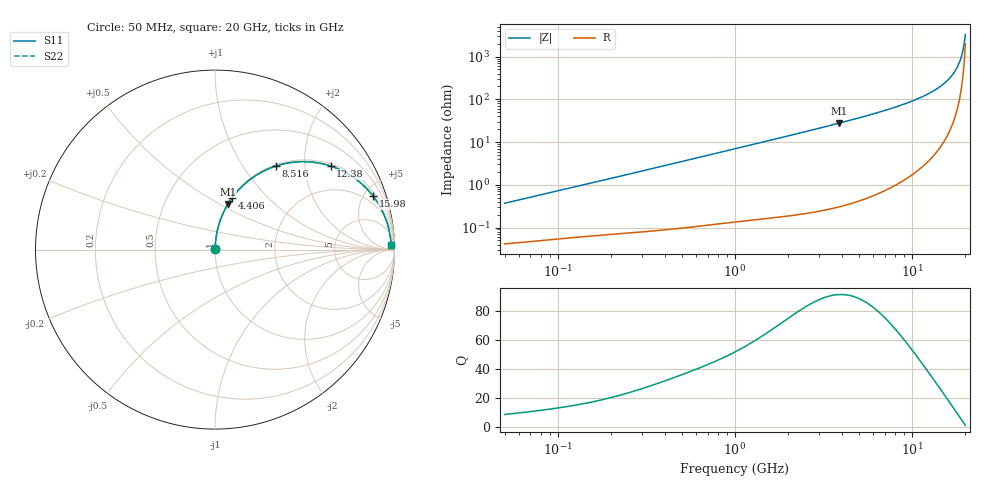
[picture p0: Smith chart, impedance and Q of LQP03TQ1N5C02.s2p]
!Murata Part Number: LQP03TQ1N5C02
!These Parameters are Measured in Series Mode Connection
!  o--[Z]--o
!Port1  Port2
!  o-------o
!Freq. Start=50[MHz] Stop=20[GHz], 401[Steps]
# Hz S RI R 50
!Freq.(Hz) S11(Real) S11(Imag) S21(Real) S21(Imag) S12(Real) S12(Imag) S22(Real) S22(Imag)
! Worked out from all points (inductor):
!   401 points, 50 MHz to 20 GHz, reference 50 ohm
!   read as one part in series: L = 1.16 nH near 51.52 MHz
!   highest Q = 91.2 at 3.85 GHz (marker M1), where L = 1.14 nH
!   S11 on the Smith chart (normalised r, x): 50 MHz: 1.00, +0.01; 4.406 GHz: 1.01, +0.64; 8.516 GHz: 1.02, +1.43; 12.38 GHz: 1.07, +2.71; 15.98 GHz: 1.31, +5.74; 20 GHz: 40, +53
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5e7  0.000427 0.00367  0.9996 -0.00367  0.9996 -0.00367  0.000427 0.00367
1.364002e8  0.000701 0.00973  0.9993 -0.00973  0.9993 -0.00973  0.000701 0.00973
3.721004e8  0.00154 0.0261  0.9985 -0.0261  0.9985 -0.0261  0.00154 0.0261
1e9  0.00616 0.0692  0.9938 -0.0692  0.9938 -0.0692  0.00616 0.0692
1.714689e9  0.0158 0.1175  0.9842 -0.1175  0.9842 -0.1175  0.0158 0.1175
2.728004e9  0.0376 0.1844  0.9624 -0.1844  0.9624 -0.1844  0.0376 0.1844
3.850025e9  0.0731 0.2549  0.9269 -0.2549  0.9269 -0.2549  0.0731 0.2549
4.405649e9  0.0951 0.2879  0.9049 -0.2879  0.9049 -0.2879  0.0951 0.2879
5.856089e9  0.1657 0.3659  0.8343 -0.3659  0.8343 -0.3659  0.1657 0.3659
7.442007e9  0.2632 0.4335  0.7368 -0.4335  0.7368 -0.4335  0.2632 0.4335
8.516016e9  0.3393 0.4657  0.6607 -0.4657  0.6607 -0.4657  0.3393 0.4657
1.050288e10  0.4943 0.49  0.5057 -0.49  0.5057 -0.49  0.4943 0.49
1.238412e10  0.6447 0.4656  0.3553 -0.4656  0.3553 -0.4656  0.6447 0.4656
1.417136e10  0.7748 0.4001  0.2252 -0.4001  0.2252 -0.4001  0.7748 0.4001
1.597544e10  0.8794 0.3001  0.1206 -0.3001  0.1206 -0.3001  0.8794 0.3001
1.721783e10  0.9308 0.2182  0.0692 -0.2182  0.0692 -0.2182  0.9308 0.2182
1.774144e10  0.9471 0.1819  0.0529 -0.1819  0.0529 -0.1819  0.9471 0.1819
1.828096e10  0.9605 0.1439  0.0395 -0.1439  0.0395 -0.1439  0.9605 0.1439
1.88369e10  0.9708 0.1046  0.0292 -0.1046  0.0292 -0.1046  0.9708 0.1046
1.912117e10  0.9748 0.0846  0.0252 -0.0846  0.0252 -0.0846  0.9748 0.0846
1.970266e10  0.9802 0.0439  0.0198 -0.0439  0.0198 -0.0439  0.9802 0.0439
2e10  0.9817 0.0234  0.0183 -0.0234  0.0183 -0.0234  0.9817 0.0234
